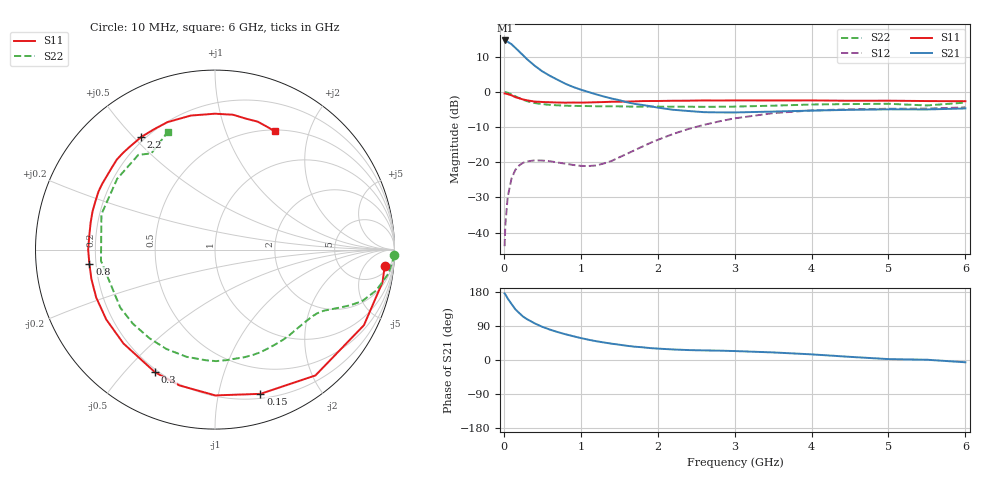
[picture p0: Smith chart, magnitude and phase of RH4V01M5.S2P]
! SIEMENS Small Signal Semiconductors
! BFR106
! Si NPN RF Bipolar Junction Transistor in SOT23
! VCE = 4 V  IC = 1.5 mA
! Common Emitter S-Parameters:  August  1996
# GHz  S  MA  R  50
!  f  S11  S21  S12  S22
! GHz  MAG  ANG  MAG  ANG  MAG  ANG  MAG  ANG
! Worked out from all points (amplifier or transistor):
!   36 points, 10 MHz to 6 GHz, reference 50 ohm
!   highest |S21| = 14.7 dB at 20 MHz (marker M1)
!   |S21| within 3 dB of that: start of sweep to 192.7 MHz
!   unconditionally stable (mu >= 1): 810.3 MHz to 1.876 GHz; 3.421 GHz to end of sweep
!   at 250 MHz: K = 0.29, MSG = 15.3 dB, |S12| = -20.1 dB
!   at 1.4 GHz: K = 1.31, MAG = 5.5 dB, |S12| = -19.6 dB
!   at 6 GHz: K = 1.02, MAG = -1.0 dB, |S12| = -4.4 dB
!   S11 on the Smith chart (normalised r, x): 10 MHz: 8, -16; 150 MHz: 0.24, -1.34; 300 MHz: 0.19, -0.61; 800 MHz: 0.17, -0.05; 2.2 GHz: 0.18, +0.53; 6 GHz: 0.52, +1.50
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0.01  0.9501 -5.6  5.404 175.8  0.0064 90.8  0.9983 -1.6
0.02  0.951 -11.0  5.405 173.1  0.0129 84.7  0.9938 -3.2
0.05  0.9306 -26.9  5.171 162.4  0.032 75.1  0.9762 -7.8
0.1  0.8971 -51.4  4.781 147.8  0.0588 62.9  0.9268 -14.2
0.15  0.8427 -72.5  4.241 133.8  0.0781 51.3  0.8697 -19.2
0.2  0.8123 -89.9  3.76 123.9  0.0902 43.4  0.8183 -22.2
0.25  0.7823 -104.7  3.328 114.6  0.0983 37.0  0.7725 -24.6
0.3  0.7606 -116.1  2.935 107.9  0.1026 32.6  0.7406 -26.4
0.4  0.7306 -134.3  2.367 96.8  0.1064 26.1  0.6967 -29.2
0.5  0.7202 -147.3  1.965 87.6  0.1058 22.9  0.6712 -31.9
0.6  0.7137 -158.1  1.696 80.1  0.1034 21.6  0.6556 -34.9
0.8  0.7042 -173.6  1.309 68.0  0.0955 23.7  0.6381 -41.7
1.1  0.7091 167.7  0.999 53.5  0.0883 39.0  0.6295 -53.1
1.6  0.7292 145.3  0.714 37.5  0.1317 68.2  0.6216 -74.8
2.2  0.75 123.3  0.558 27.8  0.2526 69.8  0.6181 -104.8
2.8  0.7555 105.1  0.512 24.7  0.3817 57.1  0.6163 -138.0
3.5  0.7571 90.0  0.526 20.0  0.4997 39.4  0.6383 -174.4
4  0.7581 82.4  0.543 14.9  0.5464 27.4  0.6627 162.7
4.5  0.7497 76.7  0.557 8.3  0.5667 17.0  0.6728 144.1
5  0.7515 71.5  0.566 2.4  0.5766 8.7  0.679 129.0
5.5  0.7425 66.5  0.564 0.7  0.5801 4.6  0.6428 123.5
6  0.7385 63.2  0.583 -6.0  0.6041 -3.3  0.7061 111.9
